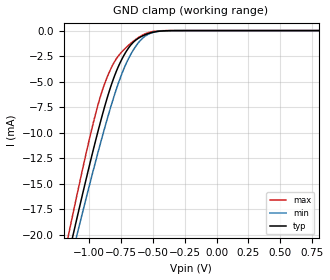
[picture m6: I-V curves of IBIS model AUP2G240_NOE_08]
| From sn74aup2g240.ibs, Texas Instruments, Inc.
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[Model]   AUP2G240_NOE_08
Model_type  Input
Vinl=0.28
Vinh=0.52
| variable   typ   min   max
C_comp   1.54pF   1.39pF   1.79pF
[Temperature Range]   40   100   -40
| Ambient temperature   25   85   -40
[Voltage range]   0.8   0.8   0.8
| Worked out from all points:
|   GND clamp passes 1 mA (typ) near -0.64 V on its own axis
[GND Clamp]
| AUP2G240_NOE_08
|   Voltage   I(typ)   I(min)   I(max)
-3.6V     -169.6mA   -161.4mA   -179.1mA
-1.165V   -22.22mA   -23.63mA   -20.26mA
-1.12V    -19.75mA   -21.32mA   -17.59mA
-1.1V     -18.67mA   -20.3mA    -16.42mA
-1.08V    -17.59mA   -19.29mA   -15.26mA
-955mV    -11.11mA   -13.14mA   -8.466mA
-855mV    -6.497mA   -8.561mA   -4.481mA
-790mV    -4.121mA   -5.903mA   -2.842mA
-720mV    -2.289mA   -3.545mA   -1.79mA
-575mV    -490.9uA   -694.4uA   -410.3uA
-400mV    -19.26uA   -23.93uA   -5.501uA
800mV     56.96pA    393.7pA    9.079pA
